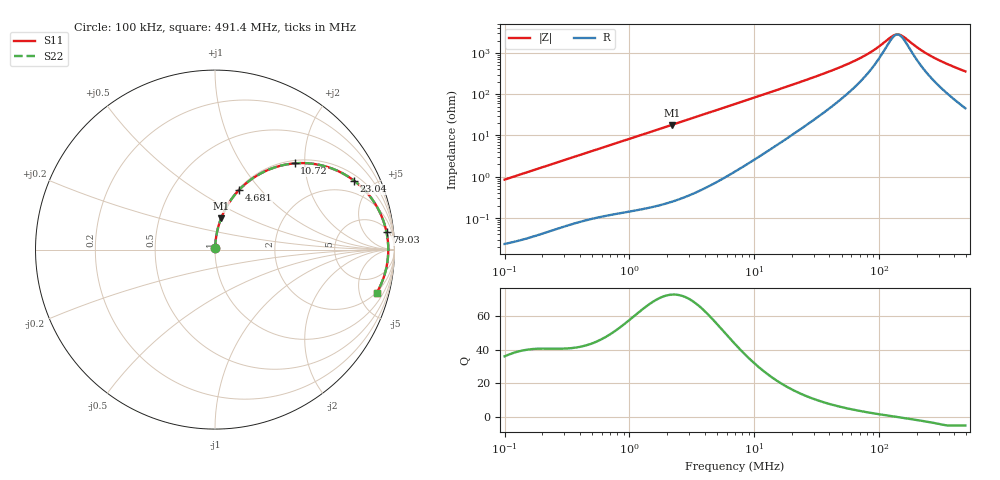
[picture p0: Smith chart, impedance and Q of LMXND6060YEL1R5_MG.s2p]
! LMXND6060YEL1R5_MG  S-PARAMETER MODEL  ( Standard Model )
! Model Generated by TAIYO YUDEN Corporation (https://www.yuden.co.jp/en/)
! Version 1.0
! TAIYO YUDEN Control No. 20240226
! Copyright(c) 2024 TAIYO YUDEN CO.,LTD. All Rights Reserved.
! Product Description (link to TY-COMPAS)
! https://ds.yuden.co.jp/TYCOMPAS/or/detail?pn=LMXND6060YEL1R5NMG&u=M
! Products Name : Inductors
! Characteristics :
!  Inductance : 1.5 [uH] , SRF(min) : 95 [MHz] , DC Resistance(max) : 0.0208 [Ohm]
!  Rated Current : Saturation  8200 [mA] , Temp Rise  4200 [mA] (40 [degC])
!  Case Size : 6.0 x 6.0 / 0.236 x 0.236 [mm/inch] , Thickness : 4.5 / 0.177 [mm/inch]
!  (Conditions: Temperature = 25 [degC] , DC Bias Current = 0 [A])
! External Node Assignments :
!  1  o---GGG---o  2
! GND o---------o GND
! Frequency Range : 0.1MHz  -  491.415554MHz  [ 402 STEP ]
# MHz S RI R 50
! Freq[MHz].  S11 Real  S11 Imag  S21 Real  S21 Imag  S12 Real  S12 Imag  S22 Real  S22 Imag
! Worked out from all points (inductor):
!   401 points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, 100 kHz to 491.4 MHz, reference 50 ohm
!   read as one part in series: L = 1.36 uH near 104.3 kHz
!   highest Q = 72.8 at 2.178 MHz (marker M1), where L = 1.31 uH
!   self-resonance near 140.4 MHz
!   S11 on the Smith chart (normalised r, x): 100 kHz: 1.00, +0.02; 4.681 MHz: 1.01, +0.77; 10.72 MHz: 1.06, +1.78; 23.04 MHz: 1.27, +3.88; 79.03 MHz: 7, +17; 491.4 MHz: 1.91, -7.08
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0.1  0.000309 0.00852  0.9997 -0.00852  0.9997 -0.00852  0.000309 0.00852
0.415258  0.00204 0.0347  0.998 -0.0347  0.998 -0.0347  0.00204 0.0347
0.911542  0.00702 0.0749  0.993 -0.0749  0.993 -0.0749  0.00702 0.0749
1.72439  0.0218 0.139  0.9782 -0.139  0.9782 -0.139  0.0218 0.139
2.178463  0.0335 0.1733  0.9665 -0.1733  0.9665 -0.1733  0.0335 0.1733
3.332136  0.0735 0.2536  0.9265 -0.2536  0.9265 -0.2536  0.0735 0.2536
4.681453  0.1341 0.3322  0.8659 -0.3322  0.8659 -0.3322  0.1341 0.3322
7.010104  0.256 0.4251  0.744 -0.4251  0.744 -0.4251  0.256 0.4251
10.72252  0.443 0.4804  0.557 -0.4804  0.557 -0.4804  0.443 0.4804
15.38805  0.6165 0.4633  0.3835 -0.4633  0.3835 -0.4633  0.6165 0.4633
23.04238  0.7755 0.3835  0.2245 -0.3835  0.2245 -0.3835  0.7755 0.3835
29.11  0.8406 0.3237  0.1594 -0.3237  0.1594 -0.3237  0.8406 0.3237
51.6672  0.9297 0.1822  0.0703 -0.1822  0.0703 -0.1822  0.9297 0.1822
79.02916  0.9557 0.0968  0.0443 -0.0968  0.0443 -0.0968  0.9557 0.0968
95.68525  0.9614 0.063  0.0386 -0.063  0.0386 -0.063  0.9614 0.063
120.8815  0.9649 0.0242  0.0351 -0.0242  0.0351 -0.0242  0.9649 0.0242
134.4321  0.9655 0.00698  0.0345 -0.00698  0.0345 -0.00698  0.9655 0.00698
149.5017  0.9654 -0.0102  0.0346 0.0102  0.0346 0.0102  0.9654 -0.0102
210.041  0.9609 -0.0664  0.0391 0.0664  0.0391 0.0664  0.9609 -0.0664
259.7707  0.9541 -0.1043  0.0459 0.1043  0.0459 0.1043  0.9541 -0.1043
357.2889  0.9353 -0.168  0.0647 0.168  0.0647 0.168  0.9353 -0.168
491.4156  0.9007 -0.2417  0.0993 0.2417  0.0993 0.2417  0.9007 -0.2417
